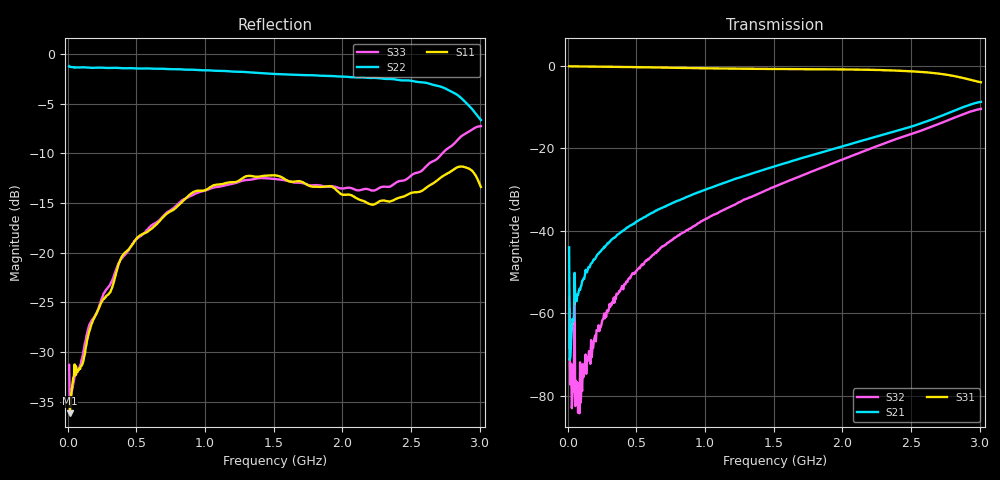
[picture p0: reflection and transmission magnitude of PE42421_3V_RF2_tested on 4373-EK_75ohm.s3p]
!Agilent Technologies,N5242A,MY49470268,A.09.90.13
!Agilent N5242A: A.09.90.13
!Date: Tuesday, October 06, 2015 13:32:04
!Correction: S11(Full 3 Port(1,2,3))
!S12(Full 3 Port(1,2,3))
!S13(Full 3 Port(1,2,3))
!S21(Full 3 Port(1,2,3))
!S22(Full 3 Port(1,2,3))
!S23(Full 3 Port(1,2,3))
!S31(Full 3 Port(1,2,3))
!S32(Full 3 Port(1,2,3))
!S33(Full 3 Port(1,2,3))
!S3P File: Measurements: <S11,S12,S13>,
!<S21,S22,S23>,
!<S31,S32,S33>:
# Hz S  dB  R 75
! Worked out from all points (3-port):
!   601 points, 10 MHz to 3.01 GHz, reference 75 ohm
!   strongest paths, dB at 10 MHz, 760 MHz, 1.51 GHz, 2.26 GHz, 3.01 GHz:
!     S31: -0.2, -0.5, -0.8, -1.1, -4.0
!     S21: -44.0, -33.3, -24.4, -17.1, -8.8
!     S32: -56.2, -42.2, -29.3, -19.4, -10.5
!   lowest |S11| = -36.2 dB at 15 MHz (marker M1), VSWR 1.03, Z = 77.3 - j0.711 ohm
!   |S11| at or under -10 dB: start of sweep to end of sweep
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1e7  -35.97 -5.0  -48.53 19.8  -0.18 -1.4
     -43.99 -132.1  -1.20 178.5  -44.23 -174.1
     -0.16 -1.3  -56.16 28.6  -31.29 -4.6
1.5e7  -36.17 -17.2  -70.58 -176.8  -0.21 -2.2
       -71.22 95.9  -1.28 178.0  -69.86 -21.2
       -0.20 -2.3  -70.80 -99.4  -34.99 -14.5
3e7  -33.75 -26.7  -67.50 83.3  -0.21 -4.5
     -63.56 79.4  -1.30 176.0  -73.12 111.7
     -0.21 -4.4  -82.93 36.7  -33.94 -29.2
7.5e7  -31.87 -45.3  -55.69 84.0  -0.22 -11.1
       -55.52 80.8  -1.33 169.9  -80.19 176.9
       -0.22 -11.1  -84.03 120.8  -31.81 -49.4
6.75e8  -16.72 174.8  -34.61 19.6  -0.49 -96.9
        -34.62 19.8  -1.46 91.1  -44.36 82.9
        -0.49 -96.9  -44.16 84.6  -16.62 179.0
1.115e9  -13.10 109.7  -28.70 -32.9  -0.71 -158.8
         -28.69 -32.7  -1.69 31.7  -35.27 24.8
         -0.72 -158.8  -35.25 25.0  -13.31 116.1
1.51e9  -12.20 52.7  -24.37 -83.1  -0.84 145.8
        -24.37 -83.2  -1.99 -24.4  -29.25 -28.8
        -0.84 145.8  -29.25 -28.6  -12.57 65.1
1.94e9  -13.46 -12.2  -20.17 -142.7  -0.92 84.1
        -20.16 -142.7  -2.21 -89.8  -23.52 -89.8
        -0.93 84.2  -23.53 -89.7  -13.32 12.1
2.375e9  -14.70 -93.5  -16.02 151.2  -1.20 19.7
         -16.01 151.3  -2.51 -157.7  -17.99 -159.5
         -1.21 19.9  -18.00 -159.4  -13.10 -45.4
3.01e9  -13.37 124.6  -8.80 16.1  -4.04 -70.0
        -8.80 16.1  -6.63 121.9  -10.50 65.1
        -4.04 -69.8  -10.51 65.3  -7.25 -166.8
